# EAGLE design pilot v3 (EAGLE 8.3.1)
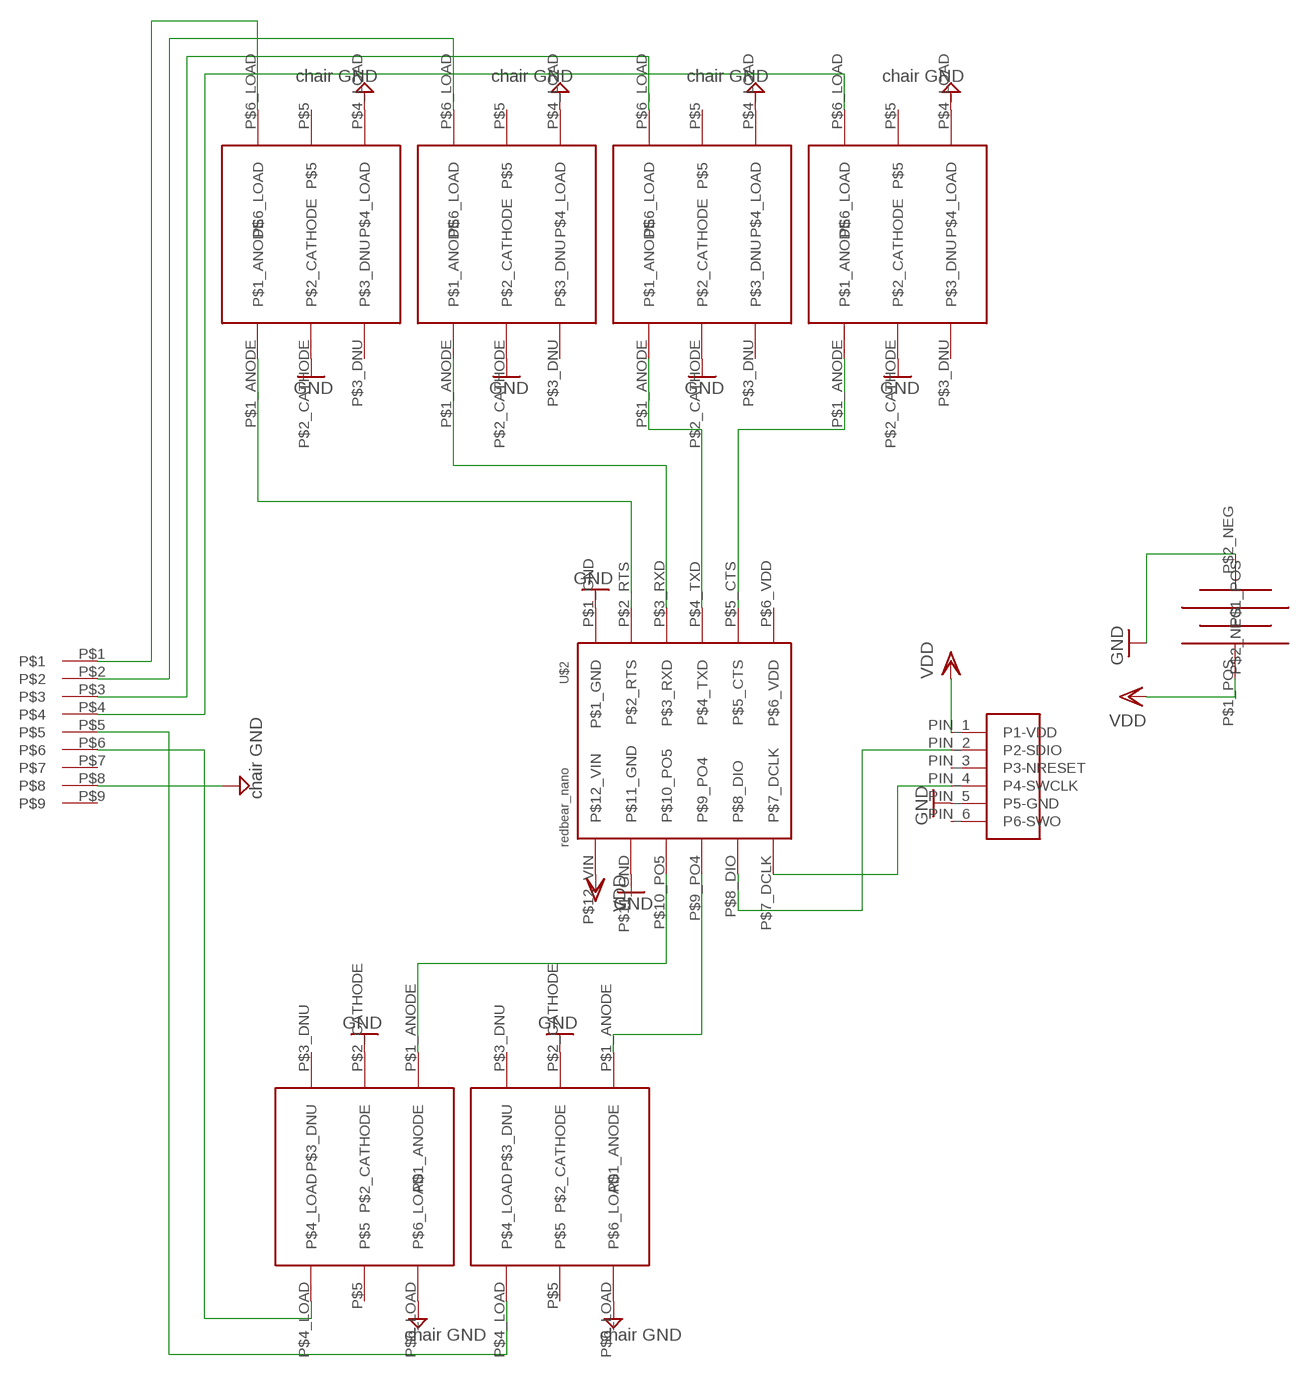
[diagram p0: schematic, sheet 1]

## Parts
U$1  TAG_CONNCET  [TAG_CONNECT]
U$2  REDBEAR_NANO  [REDBEAR_NANO]
U$3  D-SUB9PIN  [D-SUB9PIN]
U$4  VO14642AT  [VO14642AT]
U$5  VO14642AT  [VO14642AT]
U$6  VO14642AT  [VO14642AT]
U$7  VO14642AT  [VO14642AT]
U$8  VO14642AT  [VO14642AT]
U$9  KEYSTONE_1025-7  [KEYSTONE_1025-7]
U$10  VO14642AT  [VO14642AT]

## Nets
GND: U$1.PIN_5(P5-GND) U$2.P$1_GND U$2.P$11_GND U$3.P$8 U$4.P$2_CATHODE U$4.P$4_LOAD U$5.P$2_CATHODE U$5.P$6_LOAD U$6.P$2_CATHODE U$6.P$6_LOAD U$7.P$2_CATHODE U$7.P$4_LOAD U$8.P$2_CATHODE U$8.P$4_LOAD U$9.P$2_NEG U$10.P$2_CATHODE U$10.P$4_LOAD ; supply symbol labelled chair GND
N$1: U$1.PIN_4(P4-SWCLK) U$2.P$7_DCLK
N$2: U$1.PIN_2(P2-SDIO) U$2.P$8_DIO
N$4: U$3.P$5 U$5.P$4_LOAD
N$5: U$2.P$2_RTS U$8.P$1_ANODE
N$6: U$2.P$3_RXD U$7.P$1_ANODE
N$7: U$2.P$4_TXD U$10.P$1_ANODE
N$8: U$2.P$5_CTS U$4.P$1_ANODE
N$9: U$2.P$10_PO5 U$6.P$1_ANODE
N$10: U$2.P$9_PO4 U$5.P$1_ANODE
N$11: U$3.P$6 U$6.P$4_LOAD
N$12: U$3.P$4 U$4.P$6_LOAD
N$13: U$3.P$3 U$10.P$6_LOAD
N$14: U$3.P$2 U$7.P$6_LOAD
N$15: U$3.P$1 U$8.P$6_LOAD
VDD: U$1.PIN_1(P1-VDD) U$2.P$12_VIN U$9.P$1_POS
Unconnected: U$1.PIN_3(P3-NRESET) U$1.PIN_6(P6-SWO) U$2.P$6_VDD U$3.P$7 U$3.P$9 U$4.P$3_DNU U$4.P$5 U$5.P$3_DNU U$5.P$5 U$6.P$3_DNU U$6.P$5 U$7.P$3_DNU U$7.P$5 U$8.P$3_DNU U$8.P$5 U$10.P$3_DNU U$10.P$5

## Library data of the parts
U$1 = tag_connect:TAG_CONNCET
U$2 = redbearnano:REDBEAR_NANO
U$3 = d-sub 9pin:D-SUB9PIN
U$4-U$8 U$10 = vo14642at:VO14642AT: http://www.vishay.com/docs/81646/vo14642a.pdf
U$9 = coin-cell-holder:KEYSTONE_1025-7

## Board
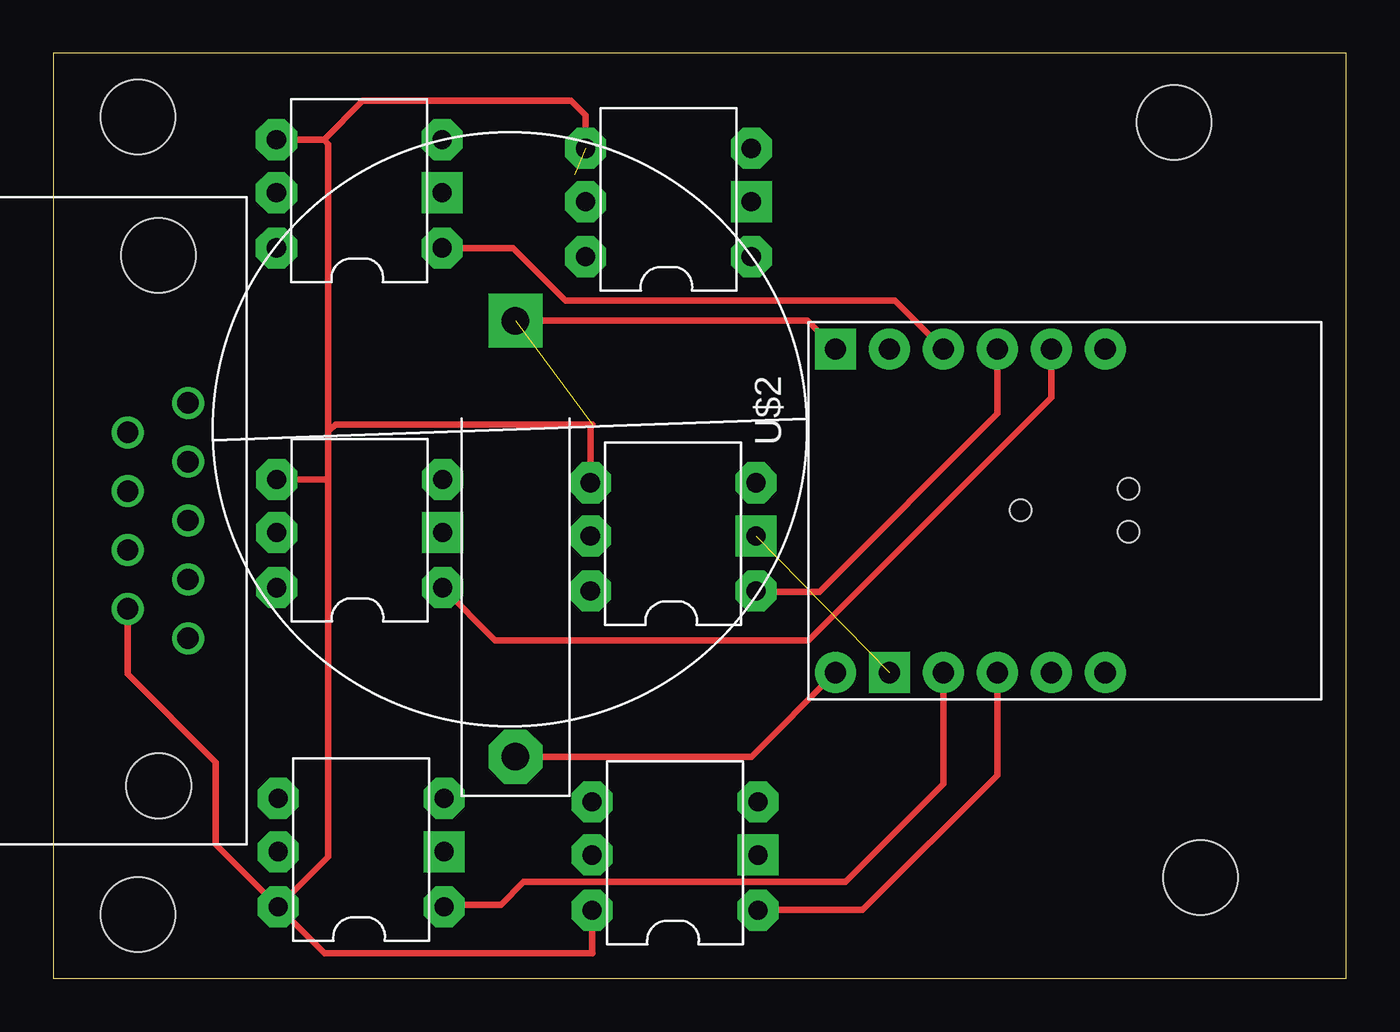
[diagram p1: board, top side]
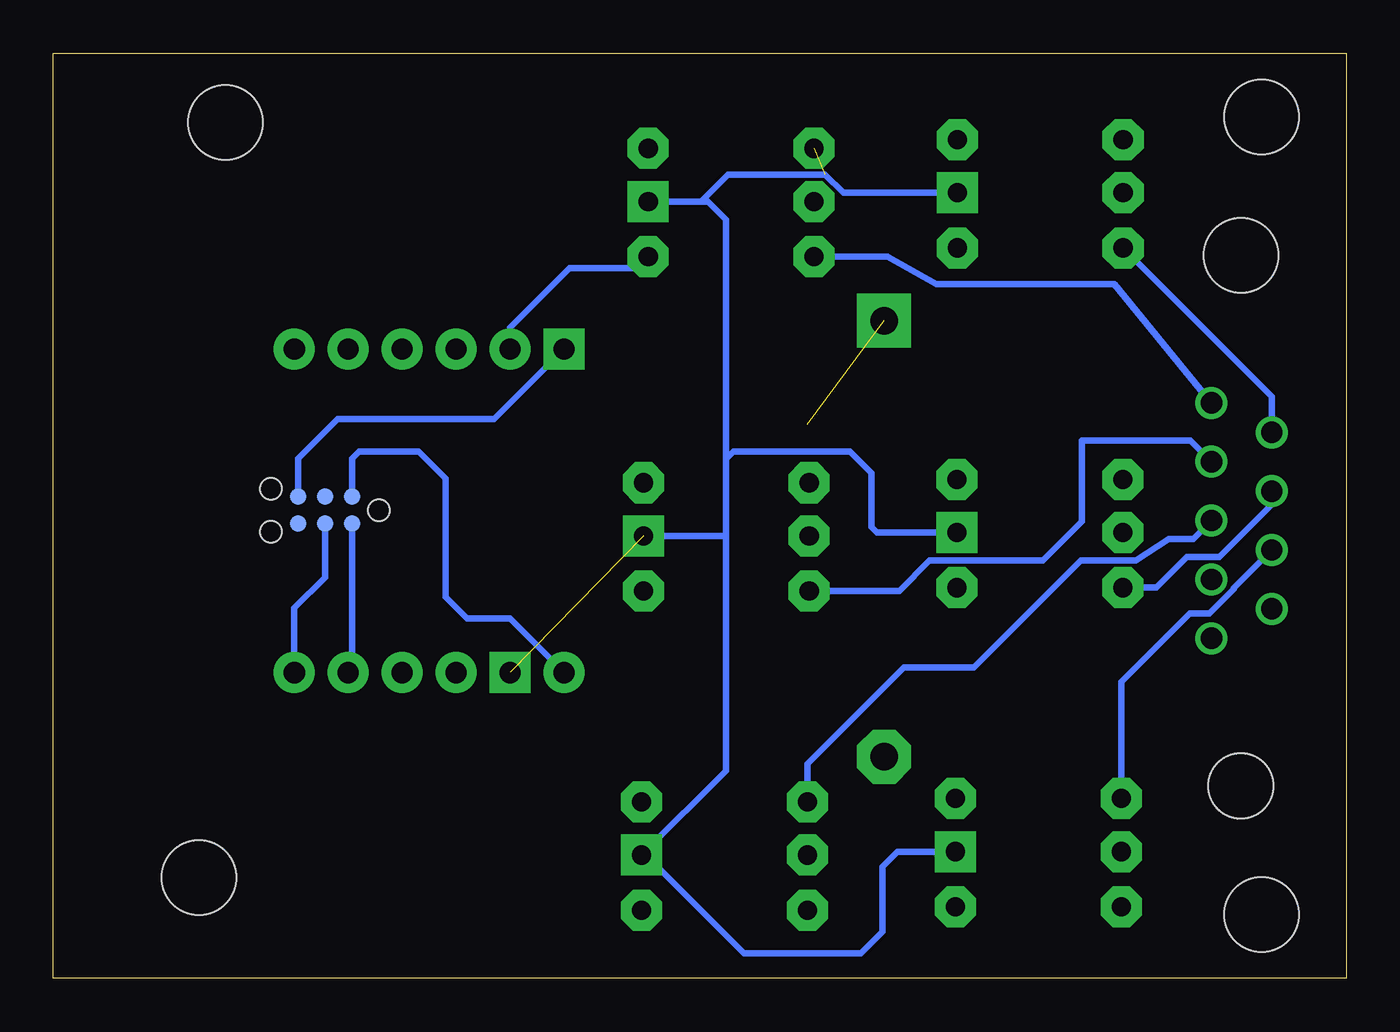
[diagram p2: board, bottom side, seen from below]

Size 60.88 x 43.57 mm. Coordinates in mm from the lower left corner, seen from the top.
Outline: 0,0 60.88,0 60.88,43.57 0,43.57 0,0
Copper layers (1*16): Top 0.035mm / dielectric 1.5mm / Bottom 0.035mm
Design rules "default": minimum track width 6mil, minimum drill 0.35mm, track to track 6mil, track to pad 6mil, pad to pad 6mil, via to via 6mil, smd to smd 6mil, copper to edge 40mil, drill to drill 6mil, minimum pad ring 10mil, minimum via ring 8mil, stop-mask expansion 4mil, vias tented up to drill 0mil, thermal gap 10mil
Holes 3.5 mm at 4,40.57 4,3 54.01,4.75 52.77,40.32

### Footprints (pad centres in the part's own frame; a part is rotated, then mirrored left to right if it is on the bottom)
TAG_CONNECT = smd 0.787 x 0.787: PIN_1 1.27,-0.635; PIN_2 1.27,0.635; PIN_3 2.54,-0.635; PIN_4 2.54,0.635; PIN_5 3.81,-0.635; PIN_6 3.81,0.635 | hole 1: 0,0; 5.08,1.016; 5.08,-1.016
REDBEAR_NANO = drill 1 pad 1.93 square: P$1_GND 0,0; P$11_GND 15.24,2.54 | drill 1 pad 1.93: P$2_RTS 0,2.54; P$3_RXD 0,5.08; P$4_TXD 0,7.62; P$5_CTS 0,10.16; P$6_VDD 0,12.7; P$7_DCLK 15.24,12.7; P$8_DIO 15.24,10.16; P$9_PO4 15.24,7.62; P$10_PO5 15.24,5.08; P$12_VIN 15.24,0
D-SUB9PIN = drill 1: P$1 0,0; P$2 1.385,-2.84; P$3 2.77,0; P$4 4.155,-2.84; P$5 5.54,0; P$6 6.925,-2.84; P$7 8.31,0; P$8 9.695,-2.84; P$9 11.08,0 | hole 3.05: 18.035,-1.385 | hole 3.5: -6.955,-1.385
VO14642AT = drill 0.9 pad 1.93 octagon: P$1_ANODE -0.7,-1.6; P$3_DNU -0.7,-6.7; P$4_LOAD 7.1,-6.7; P$5 7.1,-4.2; P$6_LOAD 7.1,-1.6 | drill 0.9 pad 1.93 square: P$2_CATHODE -0.7,-4.2
KEYSTONE_1025-7 = drill 1.3 pad 2.54 octagon: P$1_POS -1.854,0 | drill 1.3 pad 2.54 square: P$2_NEG -22.377,0

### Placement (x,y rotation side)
U$1  45.55,22.05 180 bottom
U$2  36.83,29.64 270 top
U$3  6.35,27.1 270 top
U$4  17.63,16.8 180 top
U$5  32.48,1.61 180 top
U$6  17.7,1.77 180 top
U$7  17.61,32.8 180 top
U$8  32.17,32.38 180 top
U$9  21.76,8.59 270 top
U$10  32.39,16.64 180 top

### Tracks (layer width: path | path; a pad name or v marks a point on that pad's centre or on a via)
GND  (3 unrouted)
  Top 0.305: U$3.P$8 3.51,14.33 7.66,10.18 7.66,6.31 U$6.P$6_LOAD | 12.75,39.5 U$7.P$4_LOAD | 12.75,39.5 12.95,39.29 12.95,25.74 | 12.95,25.74 12.95,23.59 | 12.95,23.59 12.95,5.73 U$6.P$6_LOAD | U$4.P$4_LOAD 12.86,23.5 12.95,23.59 | U$8.P$4_LOAD 25.07,40.64 24.38,41.32 14.57,41.32 12.75,39.5 | U$5.P$6_LOAD 25.38,1.21 25.4,1.19 12.78,1.19 U$6.P$6_LOAD | U$10.P$4_LOAD 25.29,25.97 25.4,26.08 13.29,26.08 12.95,25.74 | U$9.P$2_NEG 35.51,30.97 U$2.P$1_GND
  Bottom 0.305: U$1.PIN_5 49.36,24.48 47.5,26.34 40.13,26.34 U$2.P$1_GND | 30.37,36.58 U$8.P$2_CATHODE | 30.37,36.58 30.06,36.58 29.21,35.74 29.21,24.45 | 29.21,24.45 29.21,20.79 | 29.21,20.79 29.21,9.78 33.08,5.91 | 33.08,5.91 U$5.P$2_CATHODE | U$10.P$2_CATHODE 29.26,20.84 29.21,20.79 | U$4.P$2_CATHODE 22.09,21 22.35,21.26 22.35,23.8 23.37,24.81 28.85,24.81 29.21,24.45 | U$7.P$2_CATHODE 23.69,37 24.54,37.85 29.1,37.85 30.37,36.58 | U$6.P$2_CATHODE 21.13,5.97 21.84,5.26 21.84,2.21 22.86,1.19 28.36,1.19 33.08,5.91
N$1
  Bottom 0.305: U$1.PIN_4 48.09,18.89 49.53,17.45 U$2.P$7_DCLK
N$2
  Bottom 0.305: U$1.PIN_2 46.82,14.57 U$2.P$8_DIO
N$4
  Bottom 0.305: U$5.P$4_LOAD 25.38,10.1 20.83,14.65 17.53,14.65 13.23,18.95 | 13.23,18.95 13.21,18.97 | U$3.P$5 7.21,20.7 8.37,20.7 9.9,19.67 12.51,19.67 13.23,18.95
N$5
  Bottom 0.305: U$2.P$2_RTS 39.37,30.66 36.58,33.45 33.4,33.45 U$8.P$1_ANODE
N$6
  Top 0.305: U$7.P$1_ANODE 21.66,34.4 24.13,31.93 39.62,31.93 U$2.P$3_RXD
N$7
  Top 0.305: U$2.P$4_TXD 44.45,26.59 36.07,18.21 33.12,18.21 U$10.P$1_ANODE
N$8
  Top 0.305: U$2.P$5_CTS 46.99,27.35 35.56,15.92 20.8,15.92 U$4.P$1_ANODE
N$9
  Top 0.305: U$6.P$1_ANODE 18.51,3.48 21.08,3.48 22.15,4.54 37.29,4.54 41.91,9.16 U$2.P$10_PO5
N$10
  Top 0.305: U$2.P$9_PO4 44.45,9.57 38.1,3.22 33.19,3.22 U$5.P$1_ANODE
N$11
  Bottom 0.305: U$6.P$4_LOAD 10.6,13.96 7.37,17.19 6.45,17.19 5.29,18.35 5.29,18.39 U$3.P$6
N$12
  Bottom 0.305: U$3.P$4 3.51,22.32 5.98,19.85 7.5,19.85 8.95,18.4 U$4.P$6_LOAD
N$13
  Bottom 0.305: U$10.P$6_LOAD 21.05,18.24 19.62,19.67 14.29,19.67 12.45,21.51 12.45,25.32 7.34,25.32 U$3.P$3
N$14
  Bottom 0.305: U$3.P$2 3.51,27.4 U$7.P$6_LOAD
N$15
  Bottom 0.305: U$8.P$6_LOAD 21.62,33.98 19.3,32.69 10.92,32.69 U$3.P$1
VDD
  Top 0.305: U$9.P$1_POS 32.87,10.44 U$2.P$12_VIN
  Bottom 0.305: U$1.PIN_1 46.82,24.48 46.48,24.81 43.69,24.81 42.42,23.54 42.42,17.96 41.4,16.94 39.37,16.94 U$2.P$12_VIN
